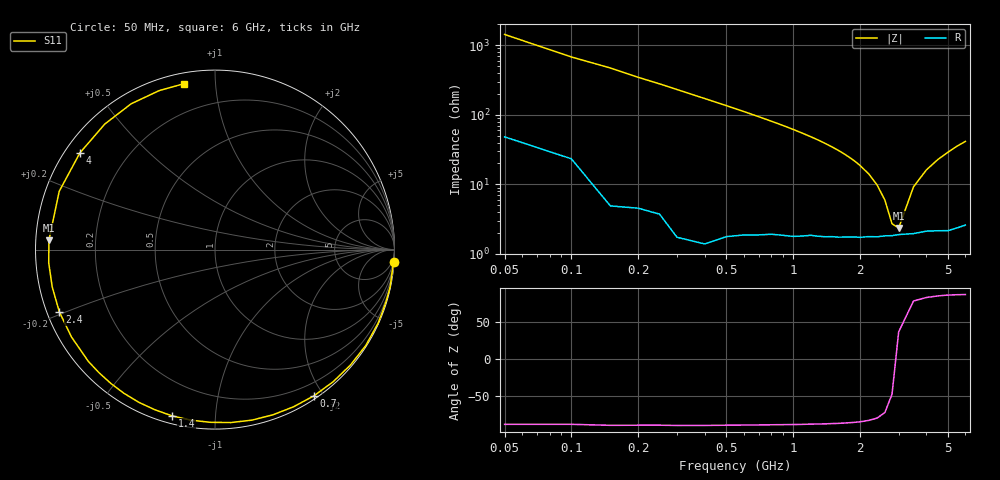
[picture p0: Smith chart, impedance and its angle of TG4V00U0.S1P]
! SIEMENS Discrete & RF Semiconductors
! BAT64
! Si Schottky Diode in SOT23
! VR = 4 V
! S-Parameters:  February  1997
# GHz  S  MA  R  50
!  f  S11
! GHz  MAG  ANG
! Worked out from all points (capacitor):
!   34 points, 50 MHz to 6 GHz, reference 50 ohm
!   read as one part to ground: C = 2.24 pF near 50 MHz
!   lowest |Z| = 2.36 ohm at 3 GHz (marker M1)
!   series resonance near 2.918 GHz, so ESL is about 1.3 nH
!   S11 on the Smith chart (normalised r, x): 50 MHz: 1, -29; 700 MHz: 0.04, -1.88; 1.4 GHz: 0.04, -0.78; 2.4 GHz: 0.04, -0.19; 4 GHz: 0.04, +0.32; 6 GHz: 0.05, +0.83
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0.05  0.9977 -4.0
0.15  0.9978 -12.1
0.2  0.9963 -16.4
0.3  0.9969 -24.4
0.4  0.9956 -32.5
0.5  0.9916 -40.4
0.6  0.9876 -48.2
0.7  0.9836 -55.9
0.8  0.979 -63.4
0.9  0.9754 -70.7
1  0.9722 -77.8
1.1  0.9676 -84.8
1.3  0.9598 -98.0
1.4  0.9568 -104.4
1.6  0.9507 -116.5
1.8  0.9448 -127.9
2  0.9412 -138.6
2.2  0.9361 -148.7
2.4  0.9342 -158.2
2.6  0.9305 -167.1
2.8  0.9293 -175.4
3  0.9268 176.8
3.5  0.9267 159.5
4  0.9256 144.4
4.5  0.9308 131.3
5  0.9372 119.9
5.5  0.9389 109.3
6  0.9402 100.6
